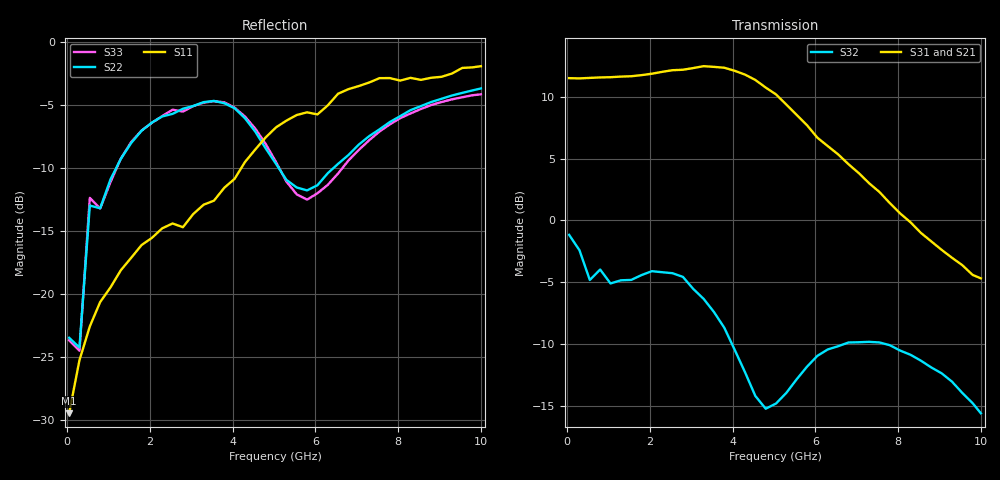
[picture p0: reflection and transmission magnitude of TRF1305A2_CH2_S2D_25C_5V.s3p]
! Created Thu Jun 26 19:36:14 2025
# hz S ma R 50
! 3 Port Network Data from SP1.SP block
! PORT[1] = INP
! PORT[2]= OUTM
! PORT[3] = OUTP
! freq  magS11  angS11  magS12  angS12  magS13  angS13
!  magS21  angS21
!  magS22  angS22  magS23  angS23
!  magS31  angS31  magS32  angS32
!  magS33  angS33
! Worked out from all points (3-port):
!   41 points, 50 MHz to 10 GHz, reference 50 ohm
!   strongest paths, dB at 50 MHz, 2.55 GHz, 5.05 GHz, 7.55 GHz, 10 GHz:
!     S31: 11.5, 12.1, 10.2, 2.3, -4.7
!     S21: 11.5, 12.2, 10.2, 2.4, -4.4
!     S32: -1.2, -4.3, -14.8, -9.9, -15.6
!   lowest |S11| = -29.4 dB at 50 MHz (marker M1), VSWR 1.07, Z = 46.8 - j0.565 ohm
!   |S11| at or under -10 dB: start of sweep to 4.212 GHz
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5e7  0.0337 -169.7  0.005918 8.2  0.0008411 138.6
     3.75 177.9  0.06713 15.4  0.8732 -0.1
     3.759 -2.2  0.8734 -0.1  0.0656 18.6
5.5e8  0.07445 -132.2  0.01284 63.1  0.009517 93.8
       3.76 159.6  0.2242 176.9  0.5908 -18.7
       3.767 -20.4  0.5735 -18.8  0.2406 175.7
1.3e9  0.1243 -125.0  0.01813 33.4  0.004918 8.7
       3.814 131.2  0.3435 109.7  0.5727 -14.5
       3.813 -48.2  0.5719 -14.2  0.3442 109.1
2.55e9  0.1905 -128.5  0.02775 22.4  0.003497 -95.9
        4.067 81.7  0.5178 54.7  0.6199 -34.0
        4.048 -97.4  0.611 -32.2  0.5379 55.2
3.3e9  0.226 -121.9  0.03768 19.0  0.01325 159.7
       4.216 48.2  0.5762 33.3  0.487 -50.5
       4.202 -131.1  0.4812 -50.7  0.5735 33.4
3.8e9  0.2639 -116.6  0.04872 6.9  0.0191 120.3
       4.163 22.8  0.5704 17.0  0.3748 -58.9
       4.141 -156.4  0.3676 -58.5  0.575 17.4
4.3e9  0.3339 -115.7  0.06288 -9.0  0.02425 78.8
       3.919 -3.2  0.4974 1.8  0.2497 -60.8
       3.885 177.7  0.2431 -57.0  0.5051 2.6
5.05e9  0.4578 -128.5  0.07588 -38.6  0.02733 26.8
        3.229 -41.0  0.3281 -4.7  0.1596 -18.3
        3.23 140.0  0.1815 -21.0  0.3334 -7.5
6.8e9  0.6486 -165.4  0.06822 -101.5  0.01587 -59.0
       1.704 -108.8  0.3557 32.0  0.3282 -14.1
       1.687 70.9  0.3205 -14.5  0.3384 35.1
1e10  0.8 146.9  0.04305 -166.6  0.005551 -151.9
      0.6009 166.5  0.6529 3.3  0.1736 -33.0
      0.5823 -17.5  0.1657 -33.9  0.6187 5.2
